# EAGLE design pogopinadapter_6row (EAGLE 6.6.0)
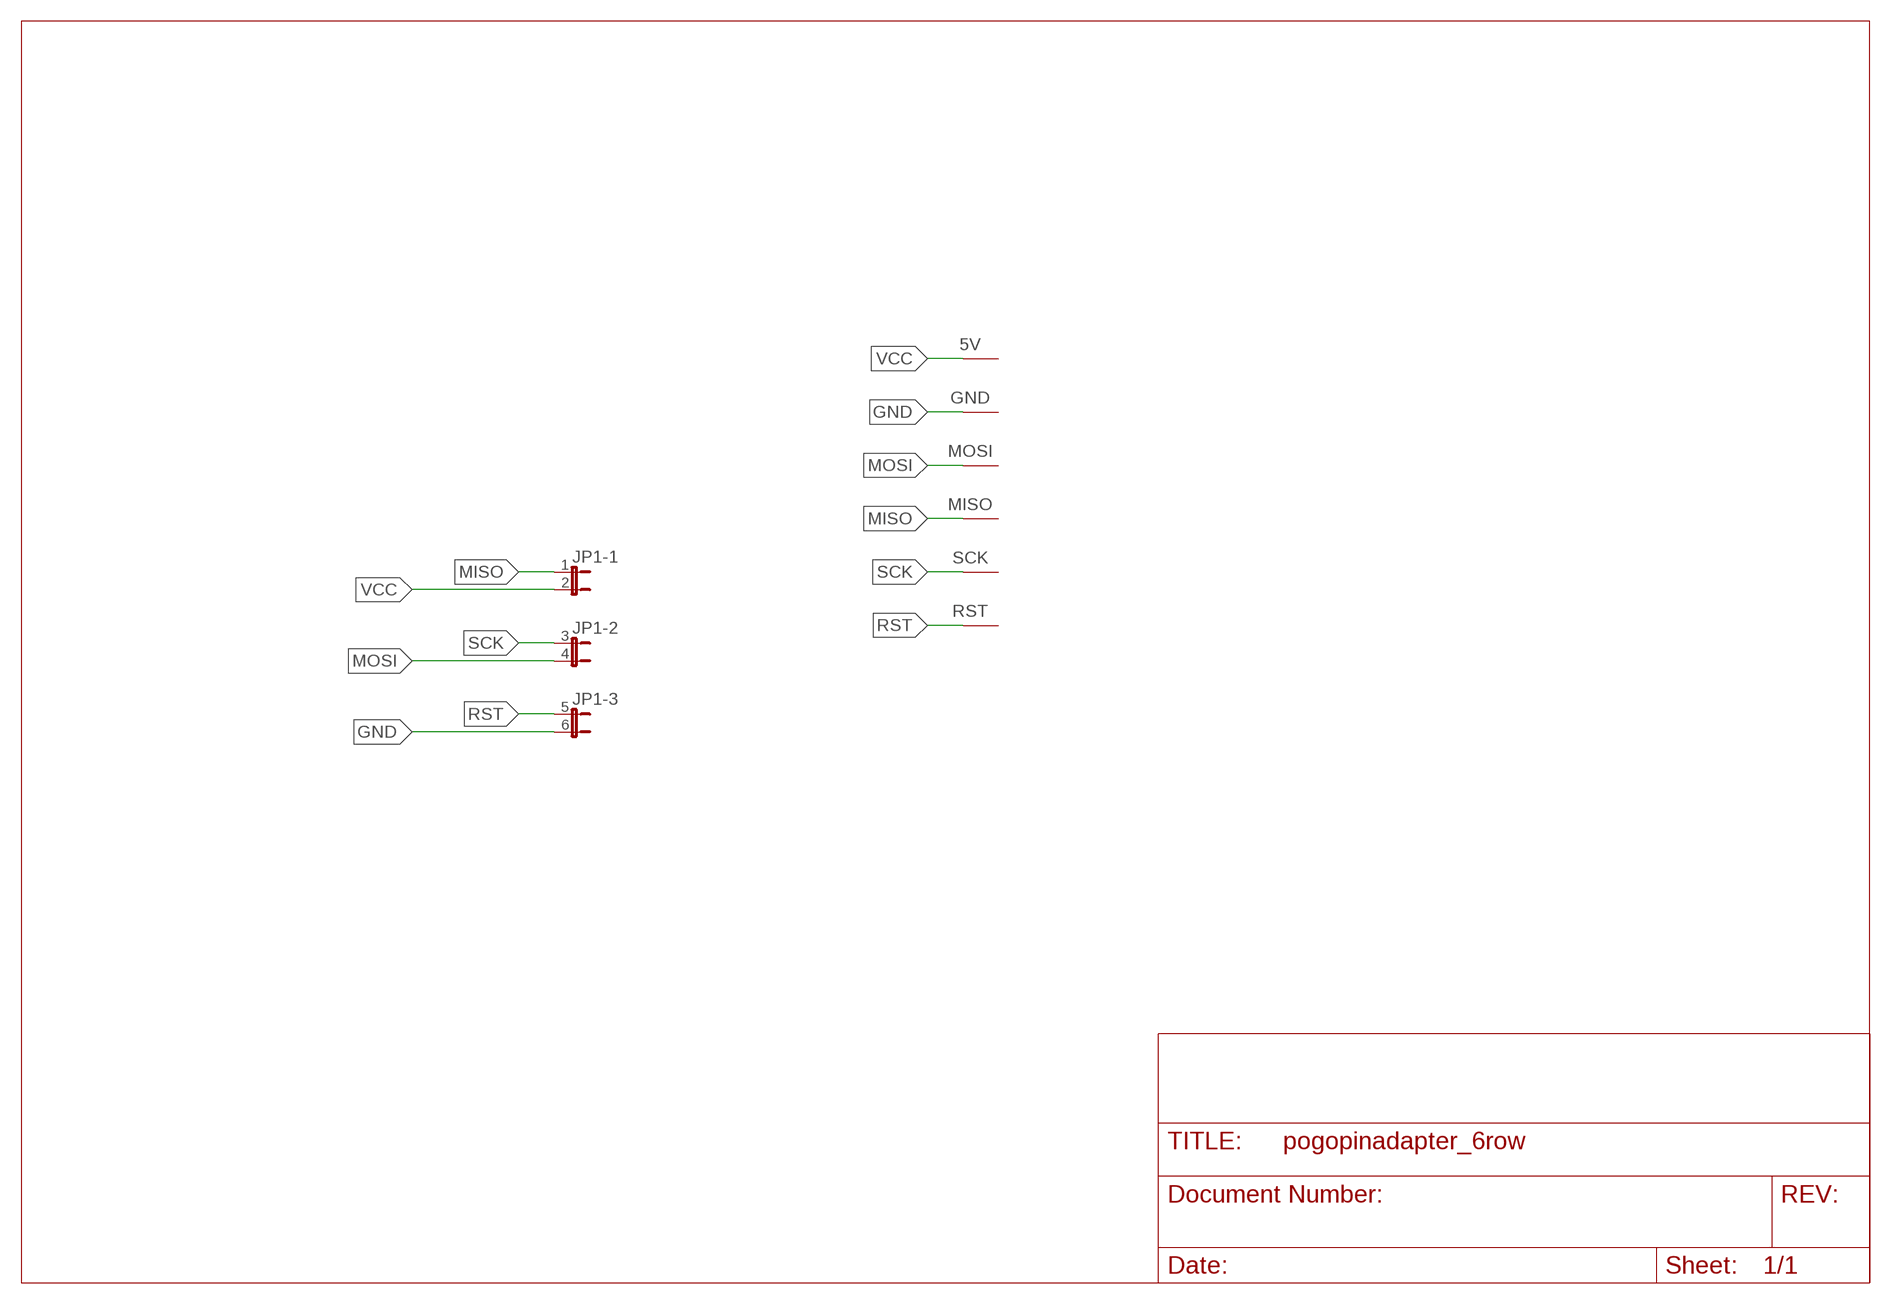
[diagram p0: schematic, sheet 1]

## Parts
5V  POGOPIN  [POGOPIN]
GND  POGOPIN  [POGOPIN]
JP1  JP3QE  [JP3Q]
MISO  POGOPIN  [POGOPIN]
MOSI  POGOPIN  [POGOPIN]
RST  POGOPIN  [POGOPIN]
SCK  POGOPIN  [POGOPIN]

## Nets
GND: GND.P$1(POGOPIN) JP1.6
MISO: JP1.1 MISO.P$1(POGOPIN)
MOSI: JP1.4 MOSI.P$1(POGOPIN)
RST: JP1.5 RST.P$1(POGOPIN)
SCK: JP1.3 SCK.P$1(POGOPIN)
VCC: 5V.P$1(POGOPIN) JP1.2

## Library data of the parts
5V GND MISO MOSI RST SCK = marco:POGOPIN
JP1 = jumper:JP3QE: JUMPER

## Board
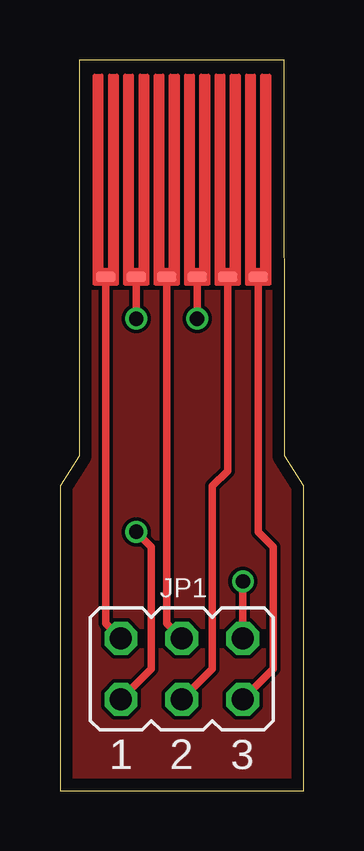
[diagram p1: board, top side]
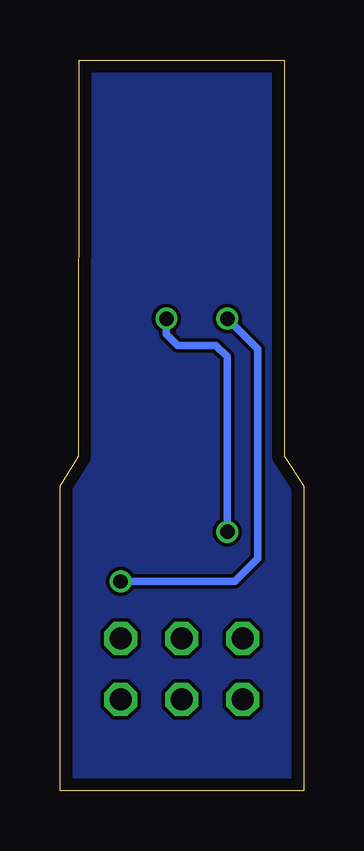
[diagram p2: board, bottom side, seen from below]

Size 10.15 x 30.47 mm. Coordinates in mm from the lower left corner, seen from the top.
Outline: 0,0 10.15,0 10.15,12.71 9.37,13.97 9.35,30.47 0.79,30.47 0.79,13.97 0,12.7 0,0
Copper layers (1*16): Top 0.035mm / dielectric 1.6mm / Bottom 0.035mm
Design rules "Elecrow_2-layer_PCB_eagle_rule": minimum track width 6mil, minimum drill 12mil, track to track 6mil, track to pad 6mil, pad to pad 6mil, via to via 8mil, smd to smd 0mil, copper to edge 20mil, drill to drill 10mil, minimum pad ring 6mil, minimum via ring 6mil, stop-mask expansion 0mil, vias tented up to drill 100mil, thermal gap 10mil

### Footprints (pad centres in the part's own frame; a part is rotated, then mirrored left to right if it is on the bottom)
POGOPIN = smd 0.813 x 0.406: P$1 0,8.414
JP3Q = drill 0.914 octagon: 1 -2.54,-1.27; 2 -2.54,1.27; 3 0,-1.27; 4 0,1.27; 5 2.54,-1.27; 6 2.54,1.27

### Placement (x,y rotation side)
5V  1.91,29.84 180 top
GND  3.17,29.84 180 top
JP1  5.08,5.08 0 top
MISO  5.71,29.84 180 top
MOSI  4.45,29.84 180 top
RST  8.26,29.84 180 top
SCK  6.99,29.84 180 top

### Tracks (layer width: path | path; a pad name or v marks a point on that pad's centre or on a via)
GND  (via drill 0.6)
  Top 0.305: JP1.6 v7.62,8.73 | v3.17,19.68 GND.P$1
  Bottom 0.305: v7.62,8.73 2.86,8.73 1.91,9.68 1.91,18.41 v3.17,19.68
MISO  (via drill 0.6)
  Top 0.305: JP1.1 3.81,5.08 3.81,10.16 v3.17,10.79 | v5.71,19.68 MISO.P$1
  Bottom 0.305: v3.17,10.79 3.17,18.1 3.65,18.57 5.24,18.57 5.71,19.05 v5.71,19.68
MOSI
  Top 0.305: JP1.4 4.45,6.99 MOSI.P$1
N$1
  pour Top: 0,0 0,12.54 0.79,13.97 0.79,30.48 9.37,30.48 9.37,13.97 10.16,12.7 10.16,0
N$2
  pour Bottom: 0,0 0,12.7 0.79,13.97 0.79,30.48 9.37,30.48 9.37,13.97 10.16,12.7 10.16,0
RST
  Top 0.305: JP1.5 8.89,5.08 8.89,10.16 8.26,10.79 RST.P$1
SCK
  Top 0.305: JP1.3 6.35,5.08 6.35,12.7 6.99,13.34 SCK.P$1
VCC
  Top 0.305: JP1.2 1.91,6.99 5V.P$1

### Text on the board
tDocu: PogoPin / adapter | by Marco / Stoffers | °
bDocu: for HK / 10A UBEC / ESC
